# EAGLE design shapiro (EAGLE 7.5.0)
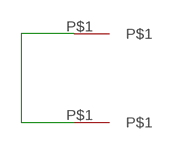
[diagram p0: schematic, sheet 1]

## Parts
U$1  SHAPIRO  [SHAPER]
U$2  SHAPIRO  [SHAPER]

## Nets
N$1: U$1.P$1 U$2.P$1

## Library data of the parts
U$1 U$2 = test160315:SHAPIRO

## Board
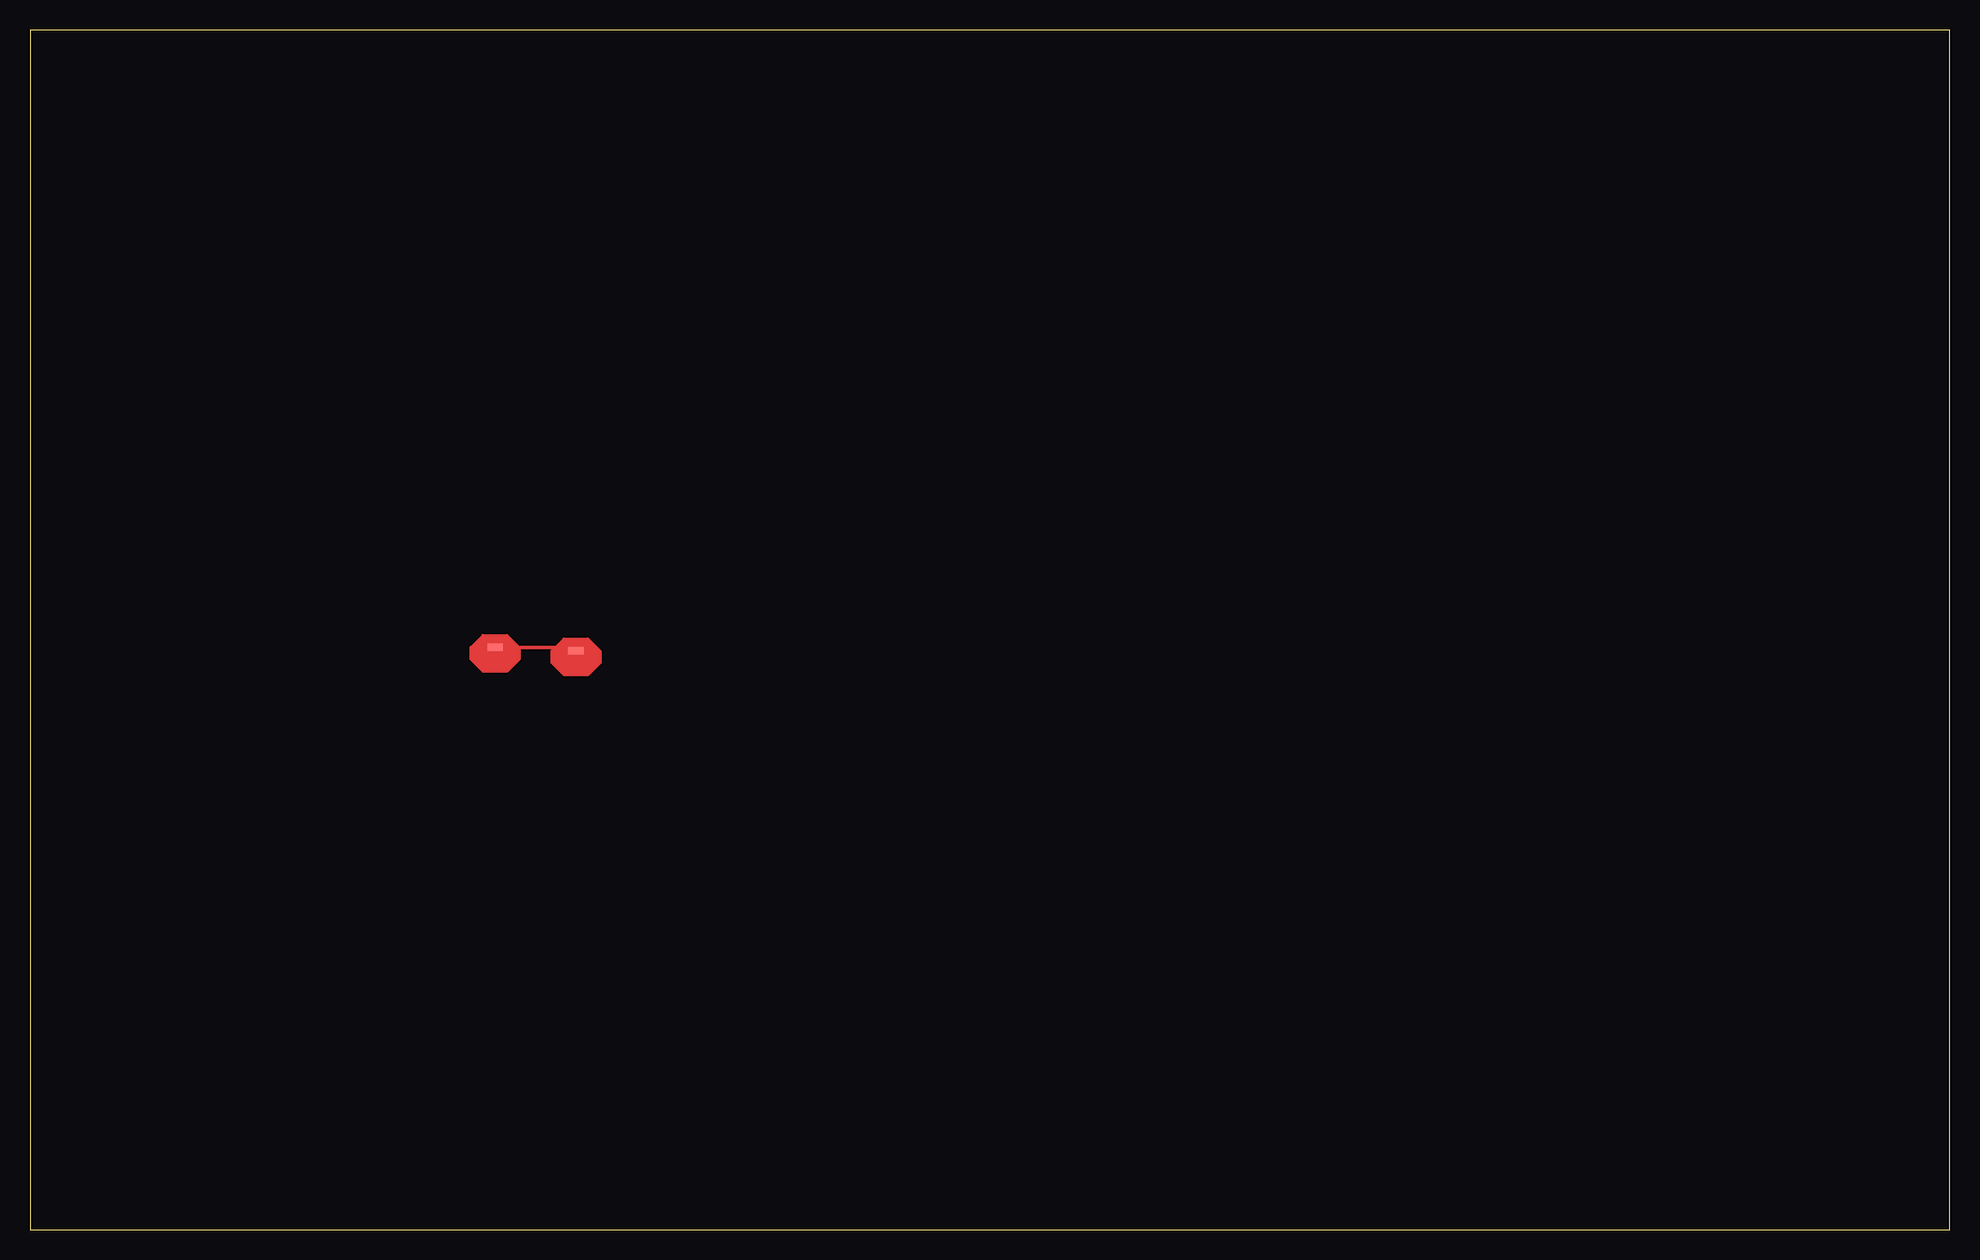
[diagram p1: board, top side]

Size 160 x 100 mm. Coordinates in mm from the lower left corner, seen from the top.
Outline: 0,0 160,0 160,100 0,100 0,0
Copper layers (1+2*3+16): Top 0.035mm / dielectric 0.5mm / Route2 0.035mm / dielectric 0.5mm / Route3 0.035mm / dielectric 0.5mm / Bottom 0.035mm
Design rules "HAREROD_4_rr200": minimum track width 0.2mm, minimum drill 0.3mm, track to track 8mil, track to pad 8mil, pad to pad 8mil, via to via 8mil, smd to smd 8mil, copper to edge 40mil, drill to drill 8mil, minimum pad ring 0.2mm, minimum via ring 0.2mm, stop-mask expansion 2mil, vias tented up to drill 0.3mm, thermal gap 0.2mm

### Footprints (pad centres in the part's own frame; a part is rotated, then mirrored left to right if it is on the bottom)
SHAPER = smd 1.27 x 0.635: P$1 0,0

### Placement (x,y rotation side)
U$1  38.76,48.54 0 top
U$2  45.5,48.25 0 top

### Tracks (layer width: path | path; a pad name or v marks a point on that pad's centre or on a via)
N$1
  Top 0.3: U$1.P$1 45.21,48.54 U$2.P$1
